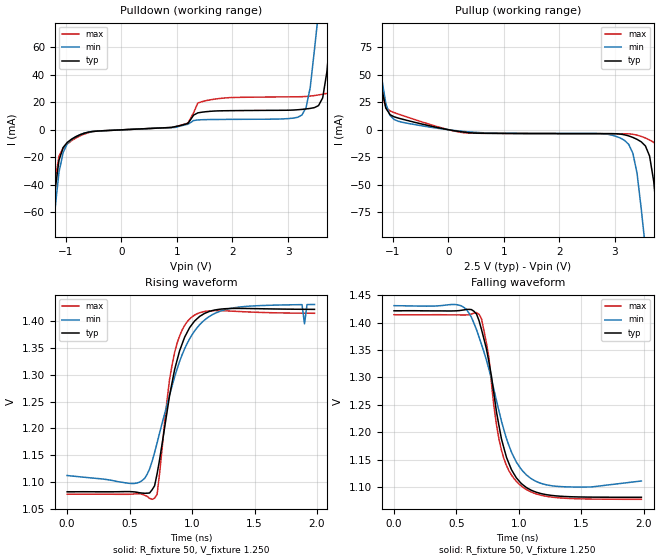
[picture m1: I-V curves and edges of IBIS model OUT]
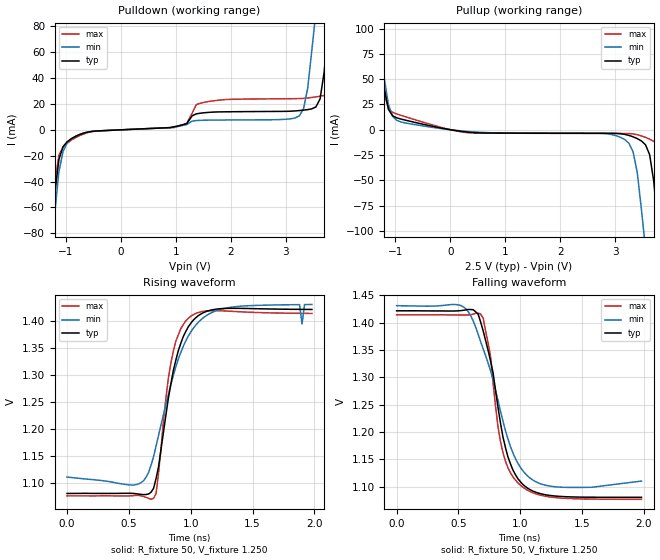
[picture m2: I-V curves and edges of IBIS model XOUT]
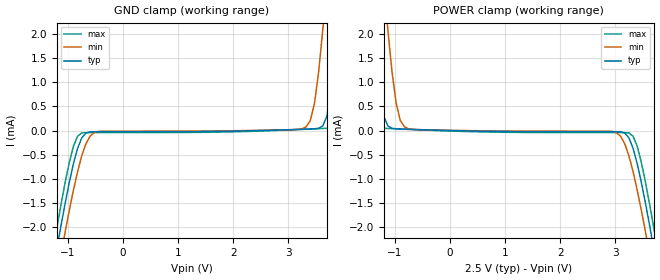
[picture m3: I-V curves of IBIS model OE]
|   IBIS File sg5032van_25v.ibs
[IBIS Ver]   3.2
[File name]   sg5032van_25v.ibs
[File Rev]   1.0
[Date]   May 1, 2013"
[Source]
[Disclaimer]
Seiko Epson Corporation makes no warranty with respect to the information
contained herein.
[Copyright]
"Copyright(C) 2013, Seiko Epson Corporation. All rights reserved."
|   Component SG5032VAN 2.5V
[Component]   sg5032van_25v
[Manufacturer]   Seiko Epson Corporation
[Package]
R_pkg   0.046   NA   NA
L_pkg   0.61n   NA   NA
C_pkg   0.95p   NA   NA
[Pin] signal_name   model_name   R_pin   L_pin   C_pin
1   OE   OE
2   GND   GND
3   GND   GND
4   OUT   OUT   0.046   0.61n   0.95p
5   XOUT   XOUT   0.046   0.61n   0.95p
6   VCC   POWER
[Diff Pin] inv_pin vdiff   tdelay_typ
4   5   0   0
| Models and submodels in the file (3): OUT (Output), XOUT (Output), OE (Input)
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[Model]   OUT
Model_type Output
Enable Active-High
Polarity Non-Inverting
Vref=1.250
Vmeas=1.250
Rref=50
Cref=0
C_comp   0.12p   0.12p   0.12p
[Temperature Range] 25   105   -40
[Voltage Range]   2.5   2.25   2.75
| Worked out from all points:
|   slope of the pulldown table from 0 to 0.375 V, typ, clamps not added: 511 ohm
|   slope of the pullup table from 0 to 0.375 V, typ, clamps not added: 139 ohm
|   falling waveform, R_fixture 50, V_fixture 1.250: 20-80 % time 171ps typ, 231ps min, 139ps max; typ from 1.42 V to 1.08 V
|   rising waveform, R_fixture 50, V_fixture 1.250: 20-80 % time 169ps typ, 258ps min, 114ps max; typ from 1.08 V to 1.42 V
[Pullup]
-2.5V     608.1mA    541.9mA    681.7mA
-1.375V   114.1mA    113.8mA    117.6mA
-1.125V   19.63mA    23.76mA    20.34mA
-900mV    10.56mA    7.689mA    14.23mA
3.175V    -4.606mA   -9.69mA    -3.648mA
3.325V    -6.999mA   -21.47mA   -4.119mA
3.55V     -14.71mA   -107.5mA   -7.473mA
3.625V    -23.87mA   -143mA     -9.269mA
3.8V      -99.16mA   -226.1mA   -15.25mA
3.95V     -179.8mA   -297.4mA   -39.81mA
4.1V      -260.6mA   -368.8mA   -125mA
5V        -746.2mA   -797.5mA   -669mA
[Pulldown]
-2.5V     -751.9mA   -683.9mA   -824.9mA
-1.3V     -98mA      -106.9mA   -93.3mA
-1.125V   -22.25mA   -31.01mA   -19.21mA
-825mV    -5.105mA   -5.185mA   -6.077mA
3.175V    14.5mA     9.051mA    23.92mA
3.325V    15.08mA    15.96mA    24.13mA
3.55V     17.52mA    85.82mA    25.25mA
3.625V    23.18mA    114.2mA    25.78mA
3.8V      85.03mA    180.3mA    27.49mA
3.95V     150.5mA    237mA      43.22mA
4.025V    183.3mA    265.4mA    76.84mA
5V        609.7mA    634.9mA    564.5mA
[Falling Waveform]
R_fixture=50
V_fixture=1.250
V_fixture_min=1.271
V_fixture_max=1.238
0s        1.422V     1.431V     1.414V
540ps     1.422V     1.43V      1.414V
680ps     1.404V     1.374V     1.415V
760ps     1.328V     1.314V     1.336V
800ps     1.269V     1.277V     1.247V
860ps     1.188V     1.22V      1.167V
940ps     1.132V     1.164V     1.122V
1.06ns    1.099V     1.122V     1.095V
1.34ns    1.083V     1.101V     1.08V
1.98ns    1.081V     1.111V     1.077V
[Rising Waveform]
R_fixture=50
V_fixture=1.250
V_fixture_min=1.271
V_fixture_max=1.238
0s        1.082V     1.112V     1.077V
560ps     1.081V     1.098V     1.078V
700ps     1.093V     1.155V     1.07V
720ps     1.115V     1.173V     1.077V
860ps     1.31V      1.296V     1.342V
1ns       1.394V     1.375V     1.408V
1.4ns     1.424V     1.427V     1.418V
1.88ns    1.422V     1.431V     1.415V
1.9ns     1.422V     1.395V     1.415V
1.98ns    1.422V     1.431V     1.415V
[Ramp]
R_load=50
dV/dt_r   2.043E-1/1.691E-10   1.915E-1/2.577E-10   2.027E-1/1.141E-10
dV/dt_f   2.042E-1/1.705E-10   1.920E-1/2.307E-10   2.021E-1/1.392E-10
|[End   OUT
[Model]   XOUT
Model_type Output
Enable Active-High
Polarity Inverting
Vref=1.250
Vmeas=1.250
Rref=50
Cref=0
C_comp   0.12p   0.12p   0.12p
[Temperature Range] 25   105   -40
[Voltage Range]   2.5   2.25   2.75
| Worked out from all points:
|   slope of the pulldown table from 0 to 0.375 V, typ, clamps not added: 511 ohm
|   slope of the pullup table from 0 to 0.375 V, typ, clamps not added: 139 ohm
|   falling waveform, R_fixture 50, V_fixture 1.250: 20-80 % time 174ps typ, 242ps min, 131ps max; typ from 1.42 V to 1.08 V
|   rising waveform, R_fixture 50, V_fixture 1.250: 20-80 % time 160ps typ, 242ps min, 111ps max; typ from 1.08 V to 1.42 V
[Pullup]
-2.5V     653.7mA    576.9mA    740.8mA
-1.375V   122.7mA    121.1mA    127.8mA
-1.125V   20.09mA    24.63mA    20.62mA
-900mV    10.59mA    7.71mA     14.28mA
3.175V    -4.613mA   -9.722mA   -3.648mA
3.325V    -7.015mA   -21.99mA   -4.125mA
3.55V     -14.85mA   -117.2mA   -7.495mA
3.625V    -24.61mA   -156.1mA   -9.299mA
3.8V      -109.4mA   -247mA     -15.33mA
3.95V     -198.8mA   -325mA     -42.68mA
4.1V      -288.3mA   -403mA     -139.8mA
5V        -826.1mA   -872mA     -750.1mA
[Pulldown]
-2.5V     -833.3mA   -748.3mA   -926mA
-1.3V     -108.2mA   -116.6mA   -104.3mA
-1.125V   -22.97mA   -32.47mA   -19.65mA
-825mV    -5.132mA   -5.203mA   -6.124mA
3.175V    14.54mA    9.083mA    24mA
3.325V    15.13mA    16.28mA    24.23mA
3.55V     17.65mA    91.32mA    25.37mA
3.625V    23.76mA    121.5mA    25.9mA
3.8V      91.41mA    191.8mA    27.66mA
3.95V     161.8mA    252.2mA    45.7mA
4.025V    197mA      282.4mA    83.55mA
5V        655.4mA    675.7mA    613.4mA
[Falling Waveform]
R_fixture=50
V_fixture=1.250
V_fixture_min=1.271
V_fixture_max=1.238
0s        1.421V     1.431V     1.414V
520ps     1.422V     1.431V     1.414V
680ps     1.401V     1.365V     1.415V
760ps     1.329V     1.312V     1.338V
820ps     1.245V     1.258V     1.209V
860ps     1.191V     1.22V      1.162V
940ps     1.131V     1.162V     1.119V
1.04ns    1.101V     1.124V     1.096V
1.3ns     1.083V     1.1V       1.08V
1.98ns    1.081V     1.111V     1.077V
[Rising Waveform]
R_fixture=50
V_fixture=1.250
V_fixture_min=1.271
V_fixture_max=1.238
0s        1.081V     1.112V     1.077V
560ps     1.081V     1.098V     1.078V
700ps     1.091V     1.15V      1.073V
840ps     1.285V     1.283V     1.323V
1ns       1.396V     1.38V      1.41V
1.42ns    1.424V     1.428V     1.417V
1.88ns    1.422V     1.431V     1.415V
1.9ns     1.422V     1.395V     1.415V
1.92ns    1.422V     1.431V     1.415V
1.98ns    1.422V     1.431V     1.415V
[Ramp]
R_load=50
dV/dt_r   2.043E-1/1.603E-10   1.916E-1/2.419E-10   2.026E-1/1.110E-10
dV/dt_f   2.042E-1/1.740E-10   1.921E-1/2.418E-10   2.021E-1/1.313E-10
|[End   XOUT
[Model]   OE
Model_type Input
Vinh=1.75
Vinl=0.75
C_comp   3p   3p   3p
[Temperature Range] 25   105   -40
[Voltage Range]   2.5   2.25   2.75
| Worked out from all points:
|   GND clamp passes 1 mA (typ) near -0.96 V on its own axis
|   POWER clamp passes 1 mA (typ) near -1.29 V on its own axis
[GND Clamp]
-2.5V     -11.65mA   -12.17mA   -11.3mA
-1.2V     -2.439mA   -3.037mA   -2.004mA
-1.05V    -1.501mA   -2.093mA   -1.07mA
-750mV    -154.2uA   -526.6uA   -49.99uA
-450mV    -23.93uA   -19.15uA   -41.66uA
3.325V    27.94uA    75.78uA    27.31uA
3.475V    35.27uA    559.6uA    34.86uA
3.625V    94.02uA    2.074mA    42.53uA
3.7V      295.2uA    2.969mA    46.51uA
3.875V    2.014mA    5.059mA    78.18uA
4.175V    5.896mA    8.645mA    2.737mA
5V        16.61mA    18.53mA    14.18mA
[POWER Clamp]
-2.5V     16.61mA    18.53mA    14.18mA
-1.675V   5.896mA    8.645mA    2.737mA
-1.375V   2.014mA    5.059mA    78.18uA
-1.2V     295.2uA    2.969mA    46.51uA
-1.125V   94.02uA    2.074mA    42.53uA
-975mV    35.27uA    559.6uA    34.86uA
-825mV    27.94uA    75.78uA    27.31uA
2.95V     -23.93uA   -19.15uA   -41.66uA
3.25V     -154.2uA   -526.6uA   -49.99uA
3.55V     -1.501mA   -2.093mA   -1.07mA
3.7V      -2.439mA   -3.037mA   -2.004mA
5V        -11.65mA   -12.17mA   -11.3mA
